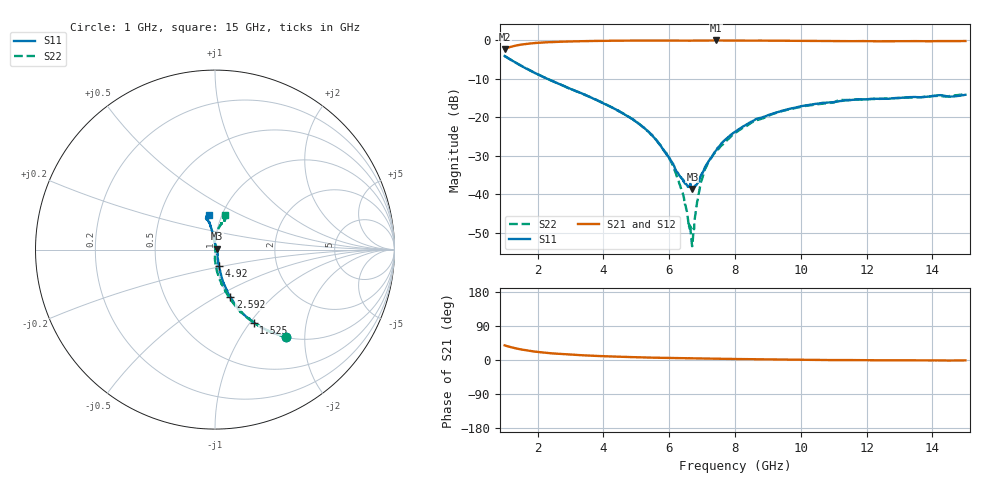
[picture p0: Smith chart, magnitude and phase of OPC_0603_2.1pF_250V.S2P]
! FILE NAME
! DATE 08/20/2012  10:43
! CORRECTED  DATA
# GHz  S  MA  R  50.00
!  FREQ  S11M  S11A  S21M  S21A  S12M  S12A  S22M  S22A
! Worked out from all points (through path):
!   1601 points, 1 GHz to 15 GHz, reference 50 ohm
!   highest |S21| = -0.06 dB at 7.423 GHz (marker M1); lowest = -2.2 dB at 1 GHz (marker M2)
!   group delay of S21, straight-line fit = 4.94 ps
!   lowest |S11| = -38.6 dB at 6.705 GHz (marker M3), VSWR 1.02, Z = 51.1 + j0.463 ohm
!   |S11| at or under -10 dB: 2.293 GHz to end of sweep
!   |S22| runs from -53.4 to -4.1 dB; largest |S21 - S12| = 0.0078
!   S11 on the Smith chart (normalised r, x): 1 GHz: 1.01, -1.61; 1.525 GHz: 1.01, -1.04; 2.592 GHz: 1.02, -0.58; 4.92 GHz: 1.03, -0.19; 15 GHz: 0.87, +0.35
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1  0.6249 -50.9  0.7735 38.7  0.7731 38.7  0.625 -50.9
1.525  0.46 -62.2  0.8837 27.5  0.8835 27.5  0.4608 -62.5
2.5925  0.278 -72.0  0.9528 16.5  0.9525 16.5  0.278 -73.4
3.33625  0.2051 -75.1  0.9719 12.6  0.9712 12.6  0.2049 -78.1
4.92  0.09236 -76.2  0.9899 7.5  0.9887 7.5  0.09288 -87.0
5.6725  0.04653 -72.1  0.9915 5.8  0.9915 5.9  0.04701 -90.7
6.1625  0.02259 -53.5  0.9891 5.0  0.9886 5.1  0.02081 -88.2
6.45125  0.01445 -21.1  0.9873 4.7  0.9867 4.7  0.008921 -72.4
6.64375  0.01382 10.6  0.9874 4.3  0.9867 4.6  0.004099 -13.2
6.705  0.01175 22.7  0.9888 4.5  0.9882 4.5  0.00214 32.7
6.74875  0.01242 32.1  0.9889 4.4  0.9888 4.4  0.003687 62.9
6.8975  0.01484 57.9  0.9907 4.2  0.9896 4.2  0.0103 89.8
7.01125  0.01899 70.1  0.9906 4.1  0.9908 4.1  0.01639 90.0
7.16  0.02527 80.5  0.9914 3.9  0.9907 3.9  0.02438 89.6
7.4225  0.03711 91.1  0.9934 3.4  0.9921 3.5  0.03621 87.0
8  0.06484 96.4  0.9909 2.7  0.99 2.7  0.06219 87.8
8.63875  0.09488 98.3  0.9882 2.1  0.9877 2.1  0.09171 83.8
9.12  0.1108 99.4  0.9861 1.5  0.9855 1.6  0.1096 82.3
10.33625  0.147 101.3  0.9803 0.3  0.9793 0.4  0.1442 76.5
11.22  0.1628 103.4  0.9713 -0.0  0.9709 0.0  0.168 74.8
12.6725  0.1741 105.4  0.9673 -0.5  0.9674 -0.5  0.1756 71.7
15  0.1963 99.4  0.9766 -1.0  0.9762 -0.9  0.2021 73.6
